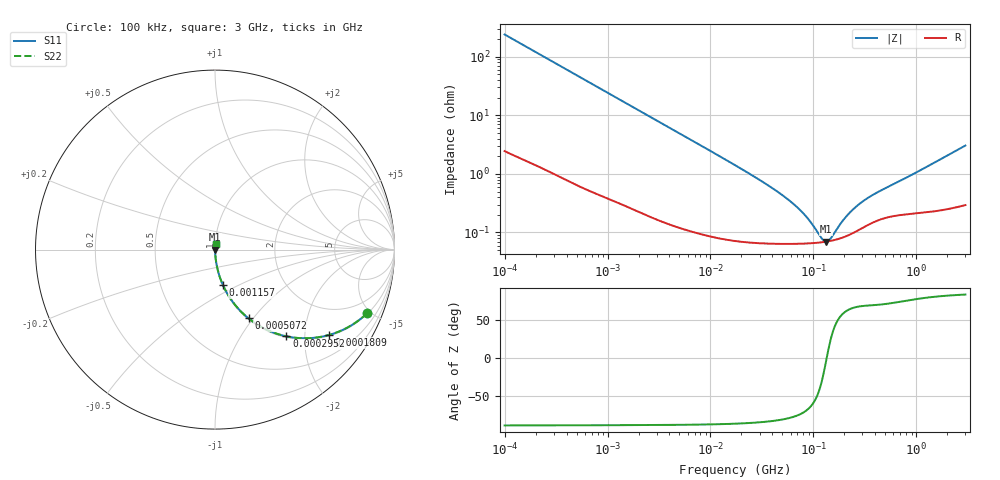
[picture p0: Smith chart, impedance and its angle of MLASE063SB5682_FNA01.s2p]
! MLASE063SB5682_FNA01  S-PARAMETER MODEL  ( Standard Model )
! Model Generated by TAIYO YUDEN Corporation (http://www.ty-top.com)
! Version 1.0
! TAIYO YUDEN Control No. 220601
! Copyright(c) 2009 TAIYO YUDEN CO.,LTD. All Rights Reserved.
! Product Description (link to TY-COMPAS)
! https://ds.yuden.co.jp/TYCOMPAS/or/detail?pn=MLASE063SB5682KFNA01&u=M
! Products Name : Multilayer Ceramic Capacitors
! Characteristics :
!  Capacitance : 6800 [pF] , Rated Voltage : 16 [V] , TCC : B / X5R
!  Case Size : 0.6 x 0.3 / 0.024 x 0.012 [mm/inch] , Thickness : 0.3 / 0.012 [mm/inch]
!  (Conditions: Temperature = 25 [degC] , DC Bias Voltage = 0 [V])
! External Node Assignments :
!  1  o---| |---o  2
! GND o---------o GND
! Frequency Range : 100kHz  -  3GHz  [ 401 STEP ]
# MHZ S RI R 50
! Freq[MHz].  S11 Real  S11 Imag  S21 Real  S21 Imag  S12 Real  S12 Imag  S22 Real  S22 Imag
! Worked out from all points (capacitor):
!   401 points, 100 kHz to 3 GHz, reference 50 ohm
!   read as one part in series: C = 6.68 nF near 105.3 kHz
!   lowest |Z| = 69.9 mohm at 132.7 MHz (marker M1)
!   series resonance near 134.7 MHz, so ESL is about 210 pH
!   S11 on the Smith chart (normalised r, x): 100 kHz: 1.05, -4.76; 180.9 kHz: 1.03, -2.64; 295.2 kHz: 1.02, -1.62; 507.2 kHz: 1.01, -0.95; 1.157 MHz: 1.01, -0.42; 3 GHz: 1.01, +0.06
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0.1  0.8472 -0.3547  0.1528 0.3547  0.1528 0.3547  0.8472 -0.3547
0.132776  0.7605 -0.4214  0.2395 0.4214  0.2395 0.4214  0.7605 -0.4214
0.180898  0.6336 -0.4761  0.3664 0.4761  0.3664 0.4761  0.6336 -0.4761
0.295187  0.3983 -0.4833  0.6017 0.4833  0.6017 0.4833  0.3983 -0.4833
0.507162  0.1868 -0.3831  0.8132 0.3831  0.8132 0.3831  0.1868 -0.3831
0.562235  0.1582 -0.3582  0.8418 0.3582  0.8418 0.3582  0.1582 -0.3582
0.786003  0.0895 -0.2782  0.9105 0.2782  0.9105 0.2782  0.0895 -0.2782
1.156955  0.0449 -0.1992  0.9551 0.1992  0.9551 0.1992  0.0449 -0.1992
3.161081  0.00751 -0.0766  0.9925 0.0766  0.9925 0.0766  0.00751 -0.0766
17.7727  0.000898 -0.0137  0.9991 0.0137  0.9991 0.0137  0.000898 -0.0137
34.73492  0.000692 -0.00666  0.9993 0.00666  0.9993 0.00666  0.000692 -0.00666
53.83243  0.000653 -0.00387  0.9993 0.00387  0.9993 0.00387  0.000653 -0.00387
75.25761  0.000648 -0.00227  0.9994 0.00227  0.9994 0.00227  0.000648 -0.00227
97.38194  0.000658 -0.00122  0.9993 0.00122  0.9993 0.00122  0.000658 -0.00122
119.6798  0.000679 -0.000437  0.9993 0.000437  0.9993 0.000437  0.000679 -0.000437
132.6759  0.000696 -5.47e-05  0.9993 5.47e-05  0.9993 5.47e-05  0.000696 -5.47e-05
147.0833  0.000719 0.000328  0.9993 -0.000328  0.9993 -0.000328  0.000719 0.000328
200.3904  0.000843 0.0015  0.9992 -0.0015  0.9992 -0.0015  0.000843 0.0015
259.3015  0.00104 0.00254  0.999 -0.00254  0.999 -0.00254  0.00104 0.00254
353.2796  0.0014 0.00382  0.9986 -0.00382  0.9986 -0.00382  0.0014 0.00382
547.5153  0.00187 0.00585  0.9981 -0.00585  0.9981 -0.00585  0.00187 0.00585
3000  0.00383 0.03  0.9962 -0.03  0.9962 -0.03  0.00383 0.03
